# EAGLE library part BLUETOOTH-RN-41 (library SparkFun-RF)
Roving Networks RN-41 Bluetooth Module The RN-41 module is a small form factor, low power, class 1 Bluetooth radio that is ideal for designers who want to add wireless capability to their products without spending significant time and money developing Bluetooth-specific hardware and software. The RN-41 supports multiple interface protocols, is simple to design in, and is fully certified, making it a complete embedded Bluetooth solution. SparkFun Products: Bluetooth SMD Module - RN-41 (WRL-12575) Bluetooth Module Breakout - Roving Networks (RN-41 v6.15) (WRL-12579)
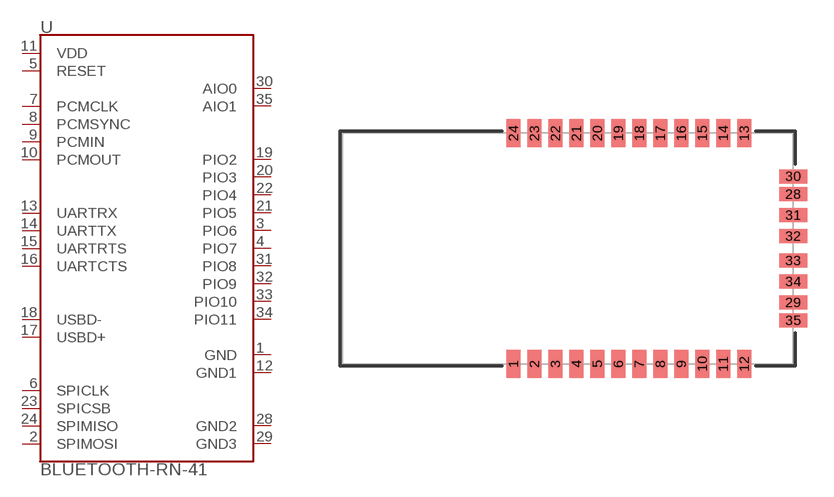
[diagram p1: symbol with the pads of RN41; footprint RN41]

Designator prefix -

## BLUETOOTH-RN-41" (PROD_ID: IC-11844; SF_ID: WRL-12575)  [RN41]
1  GND
2  SPIMOSI
3  PIO6
4  PIO7
5  RESET
6  SPICLK
7  PCMCLK
8  PCMSYNC
9  PCMIN
10  PCMOUT
11  VDD
12  GND1
13  UARTRX
14  UARTTX
15  UARTRTS
16  UARTCTS
17  USBD+
18  USBD-
19  PIO2
20  PIO3
21  PIO5
22  PIO4
23  SPICSB
24  SPIMISO
28  GND2
29  GND3
30  AIO0
31  PIO8
32  PIO9
33  PIO10
34  PIO11
35  AIO1

## Footprint RN41 (pad centres in mm)
Roving Networks RN-41 Bluetooth Module 13.4x25.8x2mm module Datasheet
smd 0.8 x 1.6: 1 -6.6,-6.6; 2 -5.4,-6.6; 3 -4.2,-6.6; 4 -3,-6.6; 5 -1.8,-6.6; 6 -0.6,-6.6; 7 0.6,-6.6; 8 1.8,-6.6; 9 3,-6.6; 10 4.2,-6.6; 11 5.4,-6.6; 12 6.6,-6.6; 13 6.6,6.6; 14 5.4,6.6; 15 4.2,6.6; 16 3,6.6; 17 1.8,6.6; 18 0.6,6.6; 19 -0.6,6.6; 20 -1.8,6.6; 21 -3,6.6; 22 -4.2,6.6; 23 -5.4,6.6; 24 -6.6,6.6
smd 1.6 x 0.8: 28 9.4,3.1; 29 9.4,-3.1; 30 9.4,4.122; 31 9.4,1.9; 32 9.4,0.7; 33 9.4,-0.7; 34 9.4,-1.9; 35 9.4,-4.122

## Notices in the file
Licensing: Creative Commons ShareAlike 4.0 International - https://creativecommons.org/licenses/by-sa/4.0
© 2015 RF Digital Corporation
